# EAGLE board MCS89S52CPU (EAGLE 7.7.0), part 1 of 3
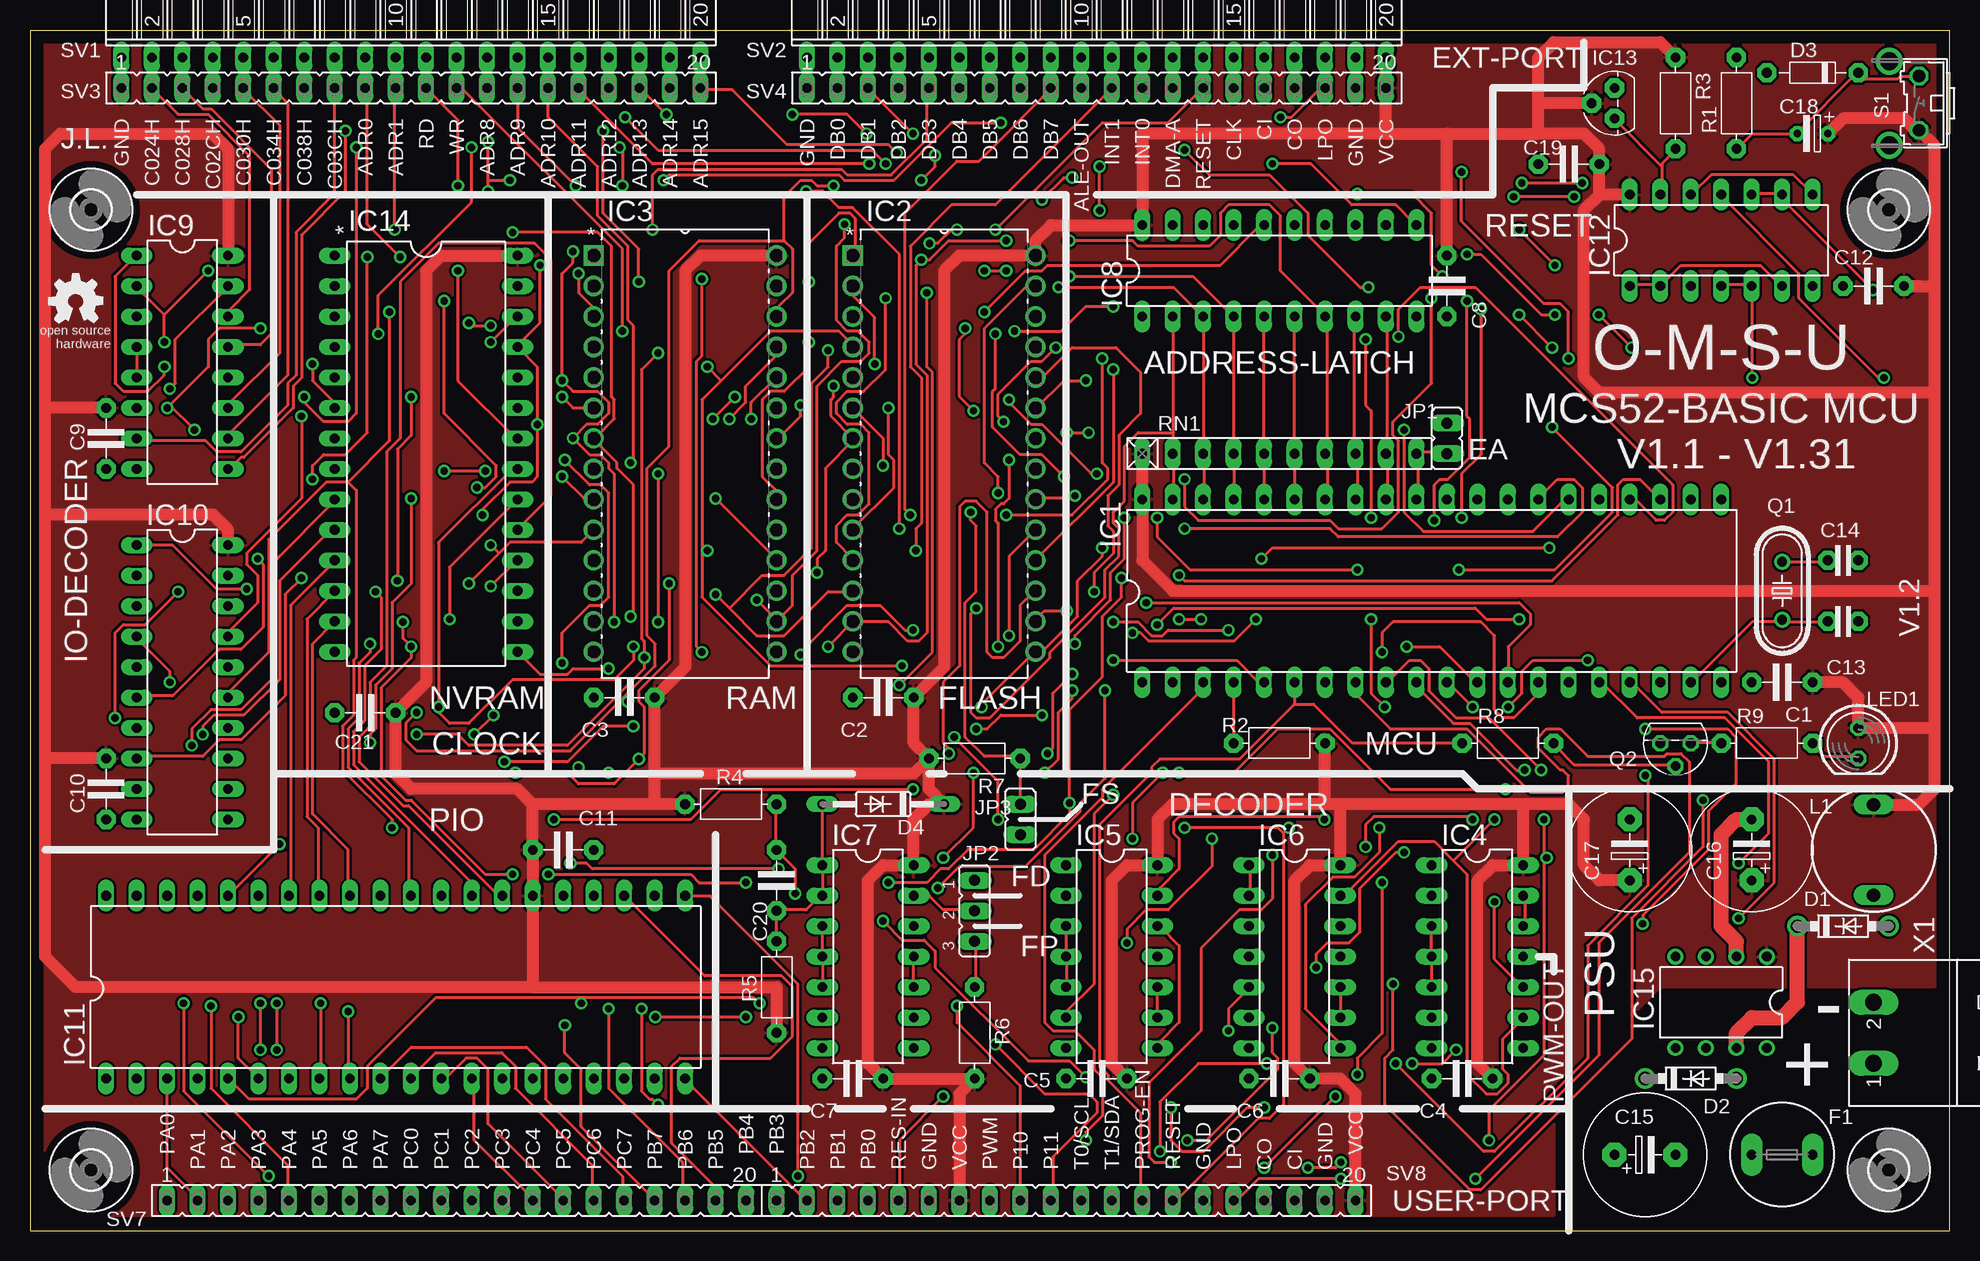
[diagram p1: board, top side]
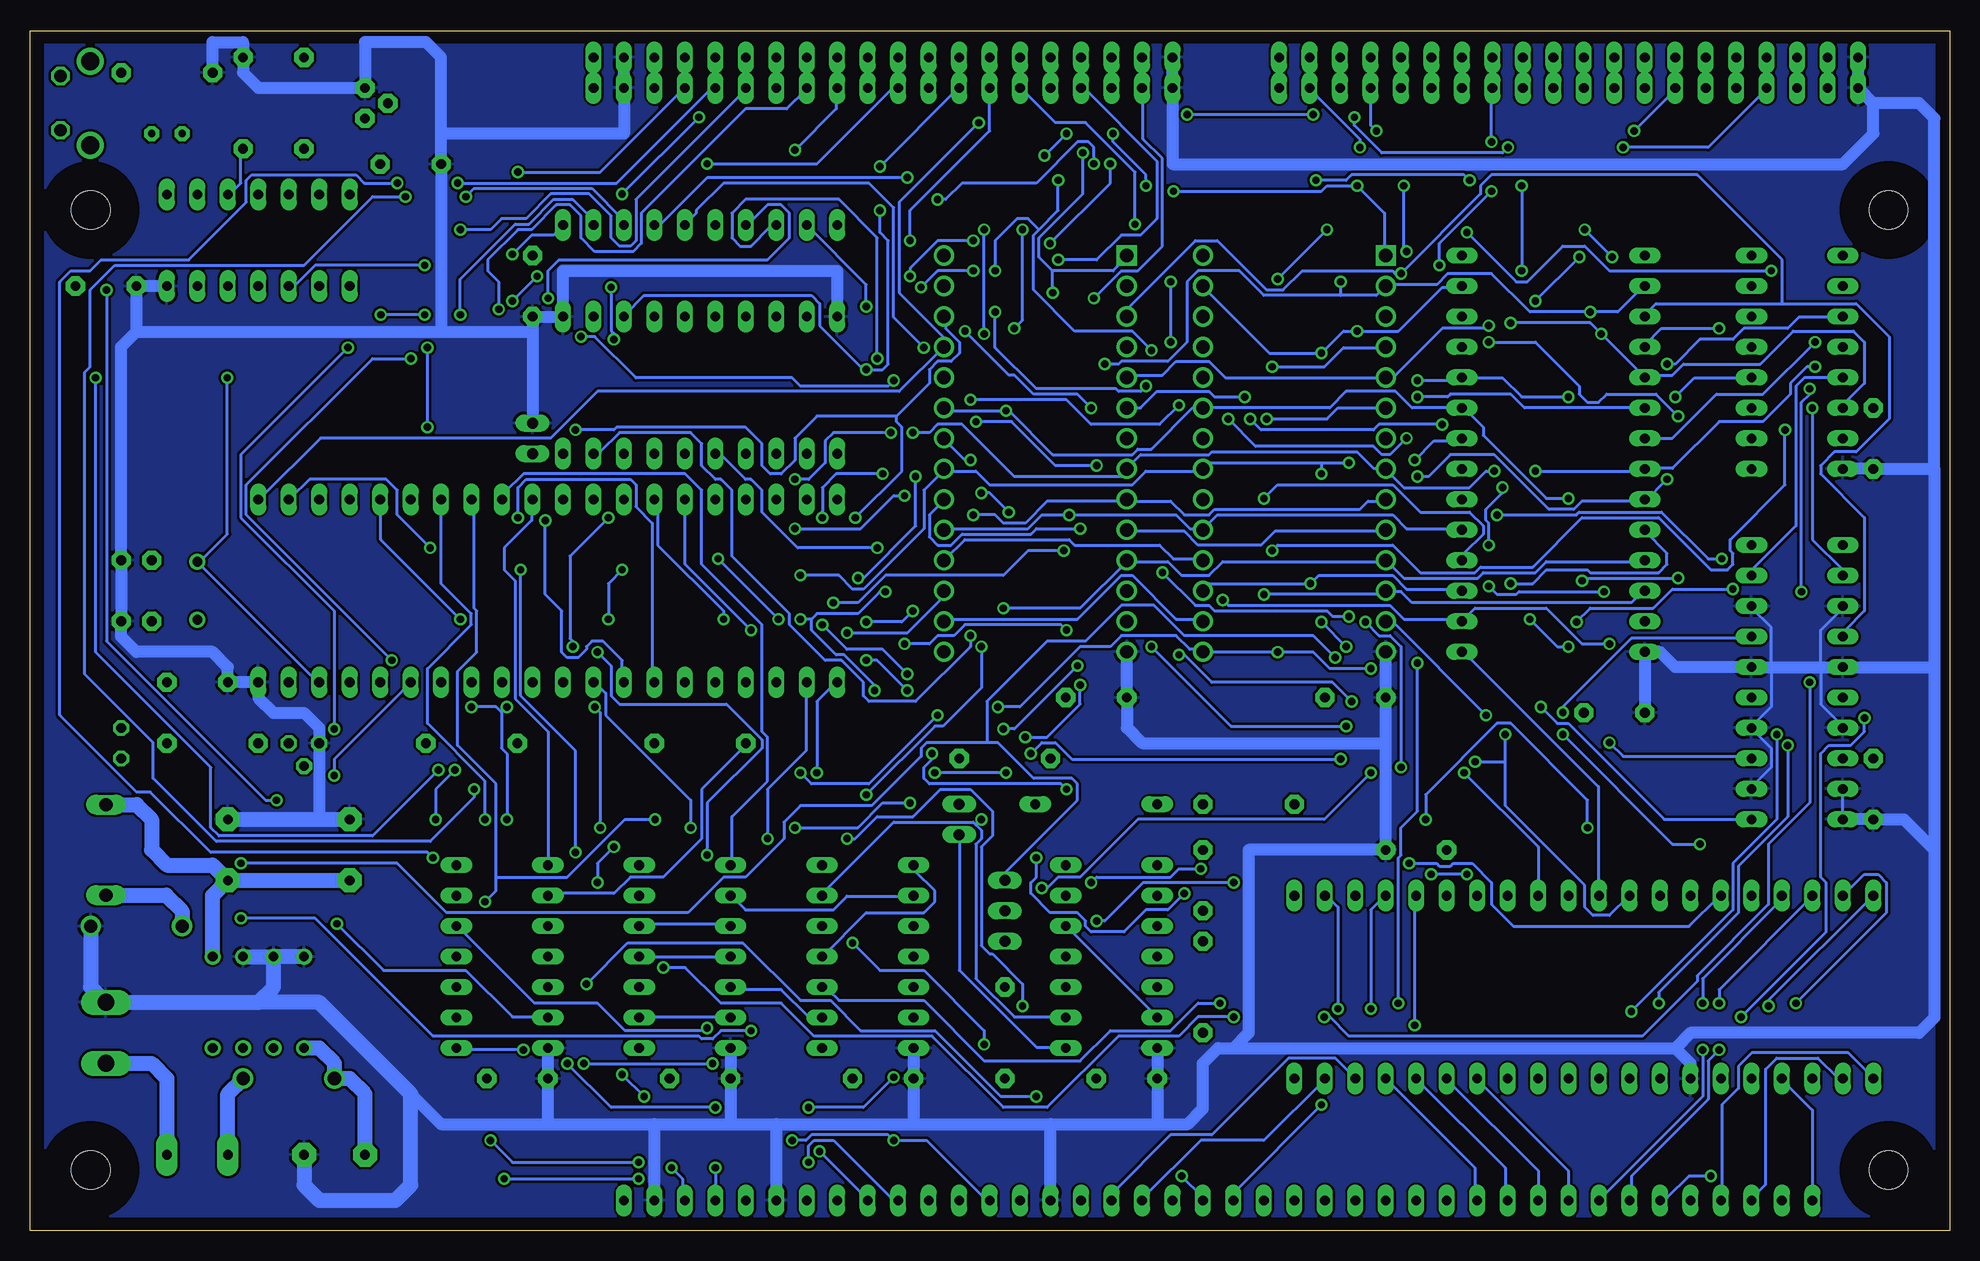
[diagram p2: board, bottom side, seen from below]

Size 160 x 100 mm. Coordinates in mm from the lower left corner, seen from the top.
Outline: 0,0 160,0 160,100 0,100 0,0
Copper layers (1*16): Top 0.035mm / dielectric 1.5mm / Bottom 0.035mm
Design rules "default": minimum track width 10mil, minimum drill 24mil, track to track 8mil, track to pad 8mil, pad to pad 8mil, via to via 8mil, smd to smd 8mil, copper to edge 40mil, drill to drill 8mil, minimum pad ring 10mil, minimum via ring 8mil, stop-mask expansion 4mil, vias tented up to drill 0mil, thermal gap 10mil

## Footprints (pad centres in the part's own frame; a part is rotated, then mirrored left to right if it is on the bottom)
C-5 = drill 0.813 pad 1.6 octagon: 1 -2.54,0; 2 2.54,0
C-2,5 = drill 0.813 pad 1.6 octagon: 1 -1.27,0; 2 1.27,0
ES-5 = drill 0.813 pad 2.007 octagon: 1 -2.54,0; 2 2.54,0
ES-2,5 = drill 0.61 pad 1.27 octagon: 1 -1.27,0; 2 1.27,0
DO41-7.6 = drill 1.1 pad 1.7: A 3.81,0; C -3.81,0
D-7,5 = drill 0.813 pad 1.6 octagon: 1 -3.81,0; 2 3.81,0
DO35-10 = drill 0.813 long: A 5.08,0; C -5.08,0
TR5 = drill 0.813 pad 1.778 long: 1 -2.54,0; 2 2.54,0
DIL40 = drill 0.813 long: 1 -24.13,-7.62; 2 -21.59,-7.62; 3 -19.05,-7.62; 4 -16.51,-7.62; 5 -13.97,-7.62; 6 -11.43,-7.62; 7 -8.89,-7.62; 8 -6.35,-7.62; 9 -3.81,-7.62; 10 -1.27,-7.62; 11 1.27,-7.62; 12 3.81,-7.62; 13 6.35,-7.62; 14 8.89,-7.62; 15 11.43,-7.62; 16 13.97,-7.62; 17 16.51,-7.62; 18 19.05,-7.62; 19 21.59,-7.62; 20 24.13,-7.62; 21 24.13,7.62; 22 21.59,7.62; 23 19.05,7.62; 24 16.51,7.62; 25 13.97,7.62; 26 11.43,7.62; 27 8.89,7.62; 28 6.35,7.62; 29 3.81,7.62; 30 1.27,7.62; 31 -1.27,7.62; 32 -3.81,7.62; 33 -6.35,7.62; 34 -8.89,7.62; 35 -11.43,7.62; 36 -13.97,7.62; 37 -16.51,7.62; 38 -19.05,7.62; 39 -21.59,7.62; 40 -24.13,7.62
DIP254P1524X482-28 = drill 1.118 square: 1 -15.24,33.02 | drill 1.118: 2 -15.24,30.48; 3 -15.24,27.94; 4 -15.24,25.4; 5 -15.24,22.86; 6 -15.24,20.32; 7 -15.24,17.78; 8 -15.24,15.24; 9 -15.24,12.7; 10 -15.24,10.16; 11 -15.24,7.62; 12 -15.24,5.08; 13 -15.24,2.54; 14 -15.24,0; 15 0,0; 16 0,2.54; 17 0,5.08; 18 0,7.62; 19 0,10.16; 20 0,12.7; 21 0,15.24; 22 0,17.78; 23 0,20.32; 24 0,22.86; 25 0,25.4; 26 0,27.94; 27 0,30.48; 28 0,33.02
DIL14 = drill 0.813 long: 1 -7.62,-3.81; 2 -5.08,-3.81; 3 -2.54,-3.81; 4 0,-3.81; 5 2.54,-3.81; 6 5.08,-3.81; 7 7.62,-3.81; 8 7.62,3.81; 9 5.08,3.81; 10 2.54,3.81; 11 0,3.81; 12 -2.54,3.81; 13 -5.08,3.81; 14 -7.62,3.81
DIL20 = drill 0.813 long: 1 -11.43,-3.81; 2 -8.89,-3.81; 3 -6.35,-3.81; 4 -3.81,-3.81; 5 -1.27,-3.81; 6 1.27,-3.81; 7 3.81,-3.81; 8 6.35,-3.81; 9 8.89,-3.81; 10 11.43,-3.81; 11 11.43,3.81; 12 8.89,3.81; 13 6.35,3.81; 14 3.81,3.81; 15 1.27,3.81; 16 -1.27,3.81; 17 -3.81,3.81; 18 -6.35,3.81; 19 -8.89,3.81; 20 -11.43,3.81
DIL16 = drill 0.813 long: 1 -8.89,-3.81; 2 -6.35,-3.81; 3 -3.81,-3.81; 4 -1.27,-3.81; 5 1.27,-3.81; 6 3.81,-3.81; 7 6.35,-3.81; 8 8.89,-3.81; 9 8.89,3.81; 10 6.35,3.81; 11 3.81,3.81; 12 1.27,3.81; 13 -1.27,3.81; 14 -3.81,3.81; 15 -6.35,3.81; 16 -8.89,3.81
TO92 = drill 0.813 pad 1.6 octagon: 1 1.27,0; 2 0,1.905; 3 -1.27,0
DIL28-6 = drill 0.813 long: 1 -16.51,-7.62; 2 -13.97,-7.62; 3 -11.43,-7.62; 4 -8.89,-7.62; 5 -6.35,-7.62; 6 -3.81,-7.62; 7 -1.27,-7.62; 8 1.27,-7.62; 9 3.81,-7.62; 10 6.35,-7.62; 11 8.89,-7.62; 12 11.43,-7.62; 13 13.97,-7.62; 14 16.51,-7.62; 15 16.51,7.62; 16 13.97,7.62; 17 11.43,7.62; 18 8.89,7.62; 19 6.35,7.62; 20 3.81,7.62; 21 1.27,7.62; 22 -1.27,7.62; 23 -3.81,7.62; 24 -6.35,7.62; 25 -8.89,7.62; 26 -11.43,7.62; 27 -13.97,7.62; 28 -16.51,7.62
DIL08 = drill 0.813 pad 1.27: 1 -3.81,-3.81; 2 -1.27,-3.81; 3 1.27,-3.81; 4 3.81,-3.81; 5 3.81,3.81; 6 1.27,3.81; 7 -1.27,3.81; 8 -3.81,3.81
JP1 = drill 0.914 long: 1 0,-1.27; 2 0,1.27
JP2 = drill 0.914 long: 1 -2.54,0; 2 0,0; 3 2.54,0
12K100-7.5 = drill 1.1 long: 1 -5.04,0; 2 2.5,0
LED5MM = drill 0.813 octagon: A -1.27,0; K 1.27,0
HC49/S = drill 0.813: 1 -2.413,0; 2 2.413,0
TO92' = drill 0.813 octagon: 1 1.27,0; 2 0,1.905; 3 -1.27,0
R-7,5 = drill 0.813 pad 1.6 octagon: 1 -3.81,0; 2 3.81,0
RN-10 = drill 0.813 long: 1 -11.43,0; 2 -8.89,0; 3 -6.35,0; 4 -3.81,0; 5 -1.27,0; 6 1.27,0; 7 3.81,0; 8 6.35,0; 9 8.89,0; 10 11.43,0
B3F-31XX = drill 1.016 octagon: 1 -2.261,-1.245; 2 2.261,-1.245 | drill 1.499 pad 2.159: 3 -3.505,1.245; 4 3.505,1.245
FE20W = drill 0.813 long: 1 -24.13,0; 2 -21.59,0; 3 -19.05,0; 4 -16.51,0; 5 -13.97,0; 6 -11.43,0; 7 -8.89,0; 8 -6.35,0; 9 -3.81,0; 10 -1.27,0; 11 1.27,0; 12 3.81,0; 13 6.35,0; 14 8.89,0; 15 11.43,0; 16 13.97,0; 17 16.51,0; 18 19.05,0; 19 21.59,0; 20 24.13,0
FE20 = drill 0.813 long: 1 -24.13,0; 2 -21.59,0; 3 -19.05,0; 4 -16.51,0; 5 -13.97,0; 6 -11.43,0; 7 -8.89,0; 8 -6.35,0; 9 -3.81,0; 10 -1.27,0; 11 1.27,0; 12 3.81,0; 13 6.35,0; 14 8.89,0; 15 11.43,0; 16 13.97,0; 17 16.51,0; 18 19.05,0; 19 21.59,0; 20 24.13,0
3,2 = hole 3.2: 0,0
MSTBA2 = drill 1.397 long: 1 -2.54,5.08; 2 2.54,5.08

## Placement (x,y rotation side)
C1  [C-5]  146.05,45.72 180 top
C2  [C-5]  71.12,44.45 180 top
C3  [C-5]  49.53,44.45 180 top
C4  [C-5]  119.38,12.7 180 top
C5  [C-5]  88.9,12.7 180 top
C6  [C-5]  104.14,12.7 180 top
C7  [C-5]  68.58,12.7 180 top
C8  [C-5]  118.11,78.74 270 top
C9  [C-5]  6.35,66.04 270 top
C10  [C-5]  6.35,36.83 270 top
C11  [C-5]  44.45,31.75 180 top
C12  [C-5]  153.67,78.74 180 top
C13  27pF  [C-2,5]  151.13,50.8 180 top
C14  27pF  [C-2,5]  151.13,55.88 180 top
C15  [ES-5]  134.62,6.35 0 top
C16  [ES-5]  143.51,31.75 90 top
C17  [ES-5]  133.35,31.75 90 top
C18  22µF  [ES-2,5]  148.59,91.44 180 top
C19  [C-5]  128.27,88.9 0 top
C20  10nF  [C-5]  62.23,29.21 270 top
C21  [C-5]  27.94,43.18 0 top
D1  1N5819  [DO41-7.6]  151.13,25.4 0 top
D2  1N5819  [DO41-7.6]  138.43,12.7 0 top
D3  [D-7,5]  148.59,96.52 0 top
D4  BAT48  [DO35-10]  71.12,35.56 180 top
F1  [TR5]  146.05,6.35 180 top
IC1  AT89S52  [DIL40]  116.84,53.34 0 top
IC2  AT28C256-15PU  [DIP254P1524X482-28]  83.82,48.26 0 top
IC3  62C256  [DIP254P1524X482-28]  62.23,48.26 0 top
IC4  74HC00N  [DIL14]  120.65,22.86 270 top
IC5  74HC00N  [DIL14]  90.17,22.86 270 top
IC6  74HC00N  [DIL14]  105.41,22.86 270 top
IC7  74HC132N  [DIL14]  69.85,22.86 270 top
IC8  74HC573N  [DIL20]  104.14,80.01 0 top
IC9  74LS138N  [DIL16]  12.7,72.39 270 top
IC10  74LS688N  [DIL20]  12.7,45.72 270 top
IC11  82C55A  [DIL40]  30.48,20.32 0 top
IC12  74LS132N  [DIL14]  140.97,82.55 0 top
IC13  TL7757  [TO92]  132.08,93.98 90 top
IC14  M48T18  [DIL28-6]  33.02,64.77 270 top
IC15  LM2574HVN-5.0  [DIL08]  140.97,19.05 180 top
JP1  [JP1]  118.11,66.04 180 top
JP2  [JP2]  78.74,26.67 270 top
JP3  [JP1]  82.55,34.29 0 top
L1  [12K100-7.5]  153.67,33.02 90 top
LED1  [LED5MM]  152.4,40.64 270 top
Q1  [HC49/S]  146.05,53.34 270 top
Q2  BC337  [TO92']  137.16,40.64 180 top
R1  1K  [R-7,5]  142.24,93.98 90 top
R2  1K  [R-7,5]  104.14,40.64 180 top
R3  1K  [R-7,5]  137.16,93.98 270 top
R4  10K  [R-7,5]  58.42,35.56 180 top
R5  15K  [R-7,5]  62.23,20.32 270 top
R6  10K  [R-7,5]  78.74,16.51 270 top
R7  10K  [R-7,5]  78.74,39.37 180 top
R8  4K7  [R-7,5]  123.19,40.64 0 top
R9  570  [R-7,5]  144.78,40.64 0 top
RN1  [RN-10]  104.14,64.77 0 top
S1  [B3F-31XX]  156.21,93.98 90 top
SV1  [FE20W]  31.75,97.79 0 top
SV2  [FE20W]  88.9,97.79 0 top
SV3  [FE20]  31.75,95.25 0 top
SV4  [FE20]  88.9,95.25 0 top
SV7  [FE20]  35.56,2.54 0 top
SV8  [FE20]  86.36,2.54 0 top
U$1  [3,2]  5.08,5.08 0 top
U$2  [3,2]  5.08,85.09 0 top
U$3  [3,2]  154.94,85.09 0 top
U$4  [3,2]  154.94,5.08 0 top
U$5  [OSHW_5MM]  3.81,77.47 0 top
X1  MSTBA2  [MSTBA2]  158.75,16.51 90 top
